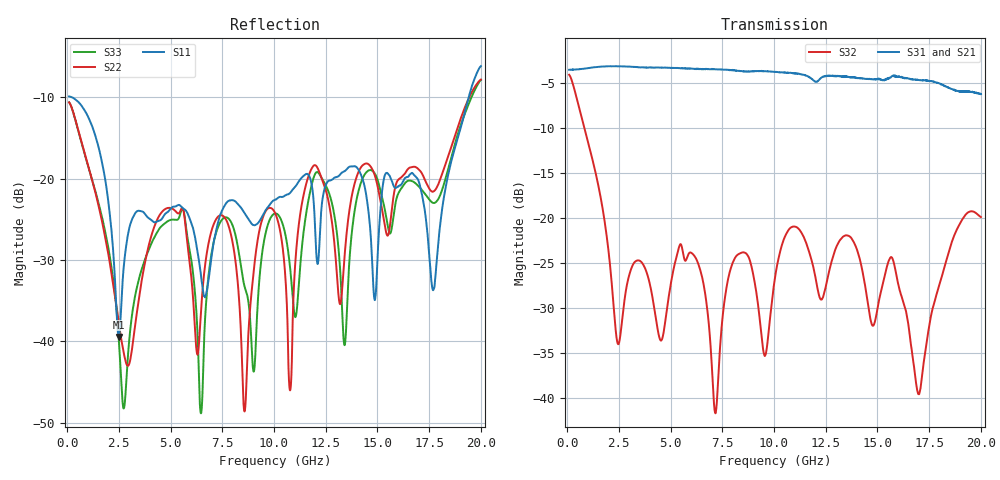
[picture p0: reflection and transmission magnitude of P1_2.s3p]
!The following data was pulled from an Agilent PNA
!This sNp file was generated from the data in the RF Test software
!NOTE:  Smoothing/Math/Corrections applied on any given trace ARE included in the data saved here
# MHz S dB R 50
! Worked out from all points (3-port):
!   6401 points, 100 MHz to 20 GHz, reference 50 ohm
!   strongest paths, dB at 100 MHz, 5.075 GHz, 10.05 GHz, 15.03 GHz, 20 GHz:
!     S31: -3.6, -3.4, -3.8, -4.6, -6.3
!     S21: -3.6, -3.4, -3.9, -4.7, -6.7
!     S32: -4.1, -26.6, -26.6, -29.8, -19.9
!   lowest |S11| = -39.4 dB at 2.5 GHz (marker M1), VSWR 1.02, Z = 49.9 + j1.06 ohm
!   |S11| at or under -10 dB: 237.5 MHz to 19.41 GHz (19.17 GHz wide, 195 % of centre)
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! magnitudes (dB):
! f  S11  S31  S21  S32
! 100 MHz  -9.9  -3.6  -3.6  -4.1
! 2.5 GHz  -39.4  -3.2  -3.2  -34.0
! 6.474 GHz  -31.9  -3.5  -3.5  -26.1
! 7.528 GHz  -23.7  -3.6  -3.6  -30.8
! 8.579 GHz  -24.3  -3.8  -3.8  -23.9
! 10.05 GHz  -22.6  -3.8  -3.9  -26.6
! 10.78 GHz  -21.8  -3.9  -4.0  -21.2
! 11.87 GHz  -21.6  -4.7  -4.8  -25.2
! 17.7 GHz  -33.7  -4.9  -4.9  -29.8
! 20 GHz  -6.2  -6.3  -6.7  -19.9
